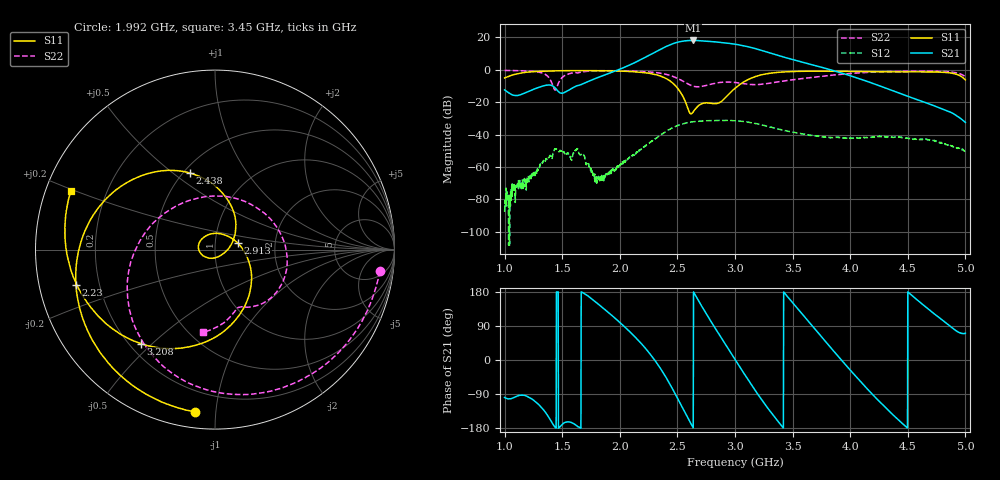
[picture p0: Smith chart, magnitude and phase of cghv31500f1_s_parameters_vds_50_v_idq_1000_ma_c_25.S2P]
!Keysight Technologies,E5071C,MY46632031,B.14.03
!Date: Fri Jul 09 16:08:55 2021
!Data & Calibration Information:
!Freq	S11:SOLT2(ON)	S21:SOLT2(ON)	S12:SOLT2(ON)	S22:SOLT2(ON)
!PortZ  Port1:50+j0  Port2:50+j0
!Above PortZ is port z conversion or system Z0 setting when saving the data.
!When reading, reference impedance value at option line is always used.
# Hz S dB R 50
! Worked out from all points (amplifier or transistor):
!   1601 points, 1 GHz to 5 GHz, reference 50 ohm
!   highest |S21| = 18.1 dB at 2.635 GHz (marker M1)
!   |S21| within 3 dB of that: 2.425 GHz to 3.056 GHz (631 MHz wide, 23 % of centre)
!   unconditionally stable (mu >= 1): start of sweep to end of sweep
!   at 1.665 GHz: K = 18.65, MAG = 5.9 dB, |S12| = -52.3 dB
!   at 3 GHz: K = 2.34, MAG = 17.1 dB, |S12| = -31.5 dB
!   at 5 GHz: K = 3167.23, MAG = -29.2 dB, |S12| = -50.0 dB
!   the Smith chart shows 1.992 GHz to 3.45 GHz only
!   S11 on the Smith chart (normalised r, x): 1.992 GHz: 0.08, -0.88; 2.23 GHz: 0.11, -0.12; 2.438 GHz: 0.54, +0.58; 2.913 GHz: 1.29, +0.09; 3.208 GHz: 0.24, -0.46; 3.45 GHz: 0.07, +0.19
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1e9  -5.02 154.2  -12.42 -98.8  -87.71 -134.6  -0.42 122.5
1.6675e9  -0.51 -15.4  -9.03 179.5  -52.22 -157.7  -1.46 55.0
1.9925e9  -0.81 -96.9  0.13 101.1  -59.49 21.8  -0.67 -7.4
2.23e9  -1.94 -165.6  7.97 28.1  -46.66 -52.2  -1.23 -57.8
2.335e9  -3.47 155.4  11.91 -14.2  -41.13 -95.9  -1.93 -87.4
2.4375e9  -6.97 107.9  15.43 -65.0  -36.57 -147.7  -3.53 -124.9
2.53e9  -14.23 53.5  17.45 -117.8  -33.69 159.2  -6.34 -169.6
2.5875e9  -23.20 -1.3  17.97 -151.1  -32.55 126.3  -8.57 155.9
2.635e9  -26.20 -102.4  18.07 -177.6  -32.13 99.3  -10.07 122.7
2.695e9  -21.54 -167.4  17.93 150.3  -31.66 66.9  -10.42 79.5
2.775e9  -20.53 140.8  17.52 109.9  -31.38 26.5  -9.18 32.7
2.84e9  -20.82 85.4  17.10 78.2  -31.29 -4.6  -8.16 3.9
2.9125e9  -17.57 15.5  16.58 43.5  -31.30 -39.2  -7.59 -21.3
3e9  -11.41 -40.9  15.75 1.6  -31.45 -81.6  -7.85 -45.2
3.105e9  -6.34 -88.6  14.33 -48.2  -32.20 -130.9  -8.85 -62.6
3.2075e9  -3.52 -128.3  12.42 -94.6  -33.62 -177.2  -9.08 -69.9
3.3175e9  -2.03 -164.6  10.05 -140.3  -35.47 137.0  -8.09 -79.5
3.45e9  -1.24 158.0  7.26 169.3  -37.73 86.8  -6.63 -98.4
3.6675e9  -0.89 104.6  3.10 90.9  -40.45 9.9  -4.73 -139.8
3.8675e9  -0.93 57.4  -0.81 19.6  -41.71 -51.1  -3.15 173.6
4.335e9  -1.28 -65.1  -12.02 -134.1  -41.42 -178.7  -1.09 62.8
5e9  -6.25 120.6  -32.43 70.8  -50.02 35.5  -4.27 -49.9
